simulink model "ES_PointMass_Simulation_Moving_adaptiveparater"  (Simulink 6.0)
settings: Solver=ode45  StartTime=0.0  StopTime=tmax  FixedStep=deltaT  MaxStep=deltaT+.001  MinStep=deltaT-.001  RelTol=1e-3
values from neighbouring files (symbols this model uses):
  ax = .05    (= 0.05)    [ES_PointMass_Values.m]    (also in ES_SimplifyPointMass_Values.m; ES_Unstable_Values.m; doublepointmass.m; pointmass.m)
  ay = .05    (= 0.05)    [ES_PointMass_Values.m]    (also in ES_SimplifyPointMass_Values.m; ES_Unstable_Values.m; doublepointmass.m; pointmass.m)
  centx = -1    [ES_PointMass_Values.m]    (also in ES_SimplifyPointMass_Values.m; ES_Unstable_Values.m; doublepointmass.m; pointmass.m)
  centy = -1    [ES_PointMass_Values.m]    (also in ES_SimplifyPointMass_Values.m; ES_Unstable_Values.m; doublepointmass.m; pointmass.m)
  cx = 20    [ES_PointMass_Values.m]    (also in ES_SimplifyPointMass_Values.m = 15; ES_Unstable_Values.m = 15; doublepointmass.m; pointmass.m)
  cy = 20    [ES_PointMass_Values.m]    (also in ES_SimplifyPointMass_Values.m = 15; ES_Unstable_Values.m = 15; doublepointmass.m; pointmass.m)
  ICx = 1    [ES_PointMass_Values.m]    (also in ES_SimplifyPointMass_Values.m; ES_Unstable_Values.m = 0; ES_Unicycle_nc_values_tune_V.m = 1.8; ES_Unicycle_nc_values_tune_V_moving.m = 1.5)
  ICy = 1    [ES_PointMass_Values.m]    (also in ES_SimplifyPointMass_Values.m; ES_Unstable_Values.m = 0; ES_Unicycle_nc_values_tune_V.m = 2; ES_Unicycle_nc_values_tune_V_moving.m = 2)
  omega = 0.1    [ES_PointMass_Values.m]    (also in ES_SimplifyPointMass_Values.m; ES_Unstable_Values.m; ES_Unicycle_Values_SI.m; abs_perturbation.m = x(:,2))
  qx = 1    [ES_PointMass_Values.m]    (also in ES_SimplifyPointMass_Values.m; ES_Unstable_Values.m; ES_Unicycle_nc_values_tune_V.m = 0.5; ES_Unicycle_nc_values_tune_V_moving.m = 0.5)
  qy = 0.5    [ES_PointMass_Values.m]    (also in ES_SimplifyPointMass_Values.m; ES_Unstable_Values.m; ES_Unicycle_nc_values_tune_V.m = 0.25; ES_Unicycle_nc_values_tune_V_moving.m = 0.25)
  root = 1    [ES_PointMass_Values.m]    (also in ES_SimplifyPointMass_Values.m; ES_Unstable_Values.m; doublepointmass.m; pointmass.m)
  tmax = 50    [ES_PointMass_Values.m]    (also in ES_SimplifyPointMass_Values.m = 80; ES_Unstable_Values.m = 20; ES_Unicycle_nc_values_tune_V.m; ES_Unicycle_nc_values_tune_V_moving.m = 300)
  wx = 30    [ES_PointMass_Values.m]    (also in ES_SimplifyPointMass_Values.m; ES_Unstable_Values.m; doublepointmass.m; pointmass.m = 20)
  wy = 30    [ES_PointMass_Values.m]    (also in ES_SimplifyPointMass_Values.m; ES_Unstable_Values.m; doublepointmass.m; pointmass.m = 20)
undefined symbols (not defined in the file or in its folder): Graph, sfunxy, simulink3, Sinks, XY
libraries: simulink x2

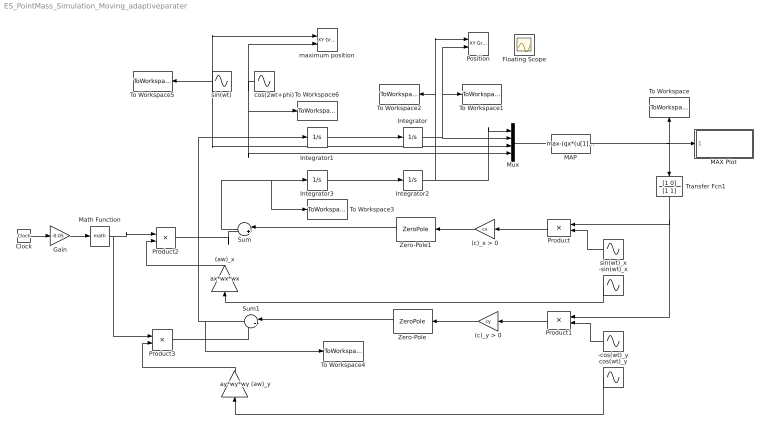
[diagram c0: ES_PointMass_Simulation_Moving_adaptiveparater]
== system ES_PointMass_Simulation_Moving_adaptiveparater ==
  (aw)_x : Gain  Orientation=up  Gain=ax*wx*wx
  (aw)_y : Gain  Orientation=up  Gain=ay*wy*wy
  (c)_x > 0 : Gain  Orientation=left  Gain=cx
  (c)_y > 0 : Gain  Orientation=left  Gain=cy
  -cos(wt)_y : Sin  Orientation=left  Amplitude=-1  Frequency=wy  Phase=pi/2  SampleTime=0
  -sin(wt)_x : Sin  Orientation=left  Frequency=wx  Phase=pi  SampleTime=0
  Clock : Clock
  Floating Scope : Scope  NumInputPorts=2
  Gain : Gain  Gain=-0.05
  Integrator : Integrator  InitialCondition=ICy
  Integrator1 : Integrator
  Integrator2 : Integrator  InitialCondition=ICx
  Integrator3 : Integrator
  MAP : Fcn  Expr=max-(qx*(u[1]-u[3])^2+qy*(u[2]-u[4])^2)^(root)
  MAX Plot : Subsystem
  Math Function : Math
  Mux : Mux
  Position : simulink/Sinks/XY Graph  xmin=centx - abs(0) -2  xmax=centx + abs(0) + 3  ymin=centy - abs(0)-2  ymax=centy + abs(0) + 3  st=-1
  Product : Product  Orientation=left
  Product1 : Product  Orientation=left
  Product2 : Product
  Product3 : Product
  Sum : Sum  Orientation=left  Inputs=|++
  Sum1 : Sum  Orientation=left  Inputs=|++
  To Workspace : ToWorkspace  VariableName=MAX  SampleTime=-1  SaveFormat=Array
  To Workspace1 : ToWorkspace  VariableName=Y  SampleTime=-1  SaveFormat=Array
  To Workspace2 : ToWorkspace  VariableName=X  SampleTime=-1  SaveFormat=Array
  To Workspace3 : ToWorkspace  VariableName=Vx  SampleTime=-1  SaveFormat=Array
  To Workspace4 : ToWorkspace  VariableName=Vy  SampleTime=-1  SaveFormat=Array
  To Workspace5 : ToWorkspace  VariableName=centerx  SampleTime=-1  SaveFormat=Array
  To Workspace6 : ToWorkspace  VariableName=centery  SampleTime=-1  SaveFormat=Array
  Transfer Fcn1 : TransferFcn  Orientation=down  Numerator=[1 0]  Denominator=[1 1]
  Zero-Pole : ZeroPole  Orientation=left  Zeros=[-2]  Poles=[-5]  Gain=[2]
  Zero-Pole1 : ZeroPole  Orientation=left  Zeros=[-2]  Poles=[-5]  Gain=[2]
  cos(2wt+phi) : Sin  Orientation=left  Frequency=2*omega  Phase=3  SampleTime=0
  cos(wt)_y : Sin  Orientation=left  Frequency=wy  Phase=pi/2  SampleTime=0
  maximum position : simulink/Sinks/XY Graph  xmin=centx - abs(0) -2  xmax=centx + abs(0) + 3  ymin=centy - abs(0)-2  ymax=centy + abs(0) + 3  st=-1
  sin(wt) : Sin  Orientation=left  Frequency=omega  SampleTime=0
  sin(wt)_x : Sin  Orientation=left  Frequency=wx  SampleTime=0
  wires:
  Integrator/1 -> To Workspace1/1, Position/2, Mux/2
  Integrator2/1 -> Mux/1, To Workspace2/1, Position/1
  Sum/1 -> Integrator3/1, To Workspace3/1
  sin(wt)_x/1 -> Product/2
  (c)_y > 0/1 -> Zero-Pole/1
  (c)_x > 0/1 -> Zero-Pole1/1
  Product1/1 -> (c)_y > 0/1
  -sin(wt)_x/1 -> (aw)_x/1
  Product/1 -> (c)_x > 0/1
  Sum1/1 -> Integrator1/1, To Workspace4/1
  Mux/1 -> MAP/1
  MAP/1 -> MAX Plot/1(MAX Seeking Value), To Workspace/1, Transfer Fcn1/1
  -cos(wt)_y/1 -> Product1/2
  cos(wt)_y/1 -> (aw)_y/1
  Transfer Fcn1/1 -> Product/1, Product1/1
  Integrator1/1 -> Integrator/1
  Integrator3/1 -> Integrator2/1
  Zero-Pole/1 -> Sum1/1
  Zero-Pole1/1 -> Sum/1
  sin(wt)/1 -> maximum position/1, To Workspace5/1, Mux/3
  cos(2wt+phi)/1 -> maximum position/2, To Workspace6/1, Mux/4
  Product2/1 -> Sum/2
  (aw)_y/1 -> Product3/2
  Product3/1 -> Sum1/2
  (aw)_x/1 -> Product2/2
  Clock/1 -> Gain/1
  Gain/1 -> Math Function/1
  Math Function/1 -> Product2/1, Product3/1

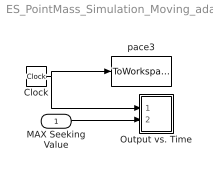
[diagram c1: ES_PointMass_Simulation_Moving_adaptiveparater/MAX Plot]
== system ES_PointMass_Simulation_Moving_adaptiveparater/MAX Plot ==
  MAX Seeking Value : Inport  Port=1  LatchInput=off
  Clock : Clock
  Output vs. Time : Subsystem  AncestorBlock=simulink3/Sinks/XY Graph  LoadFcn=sfunxy([],[],[],'LoadBlock')  StartFcn=sfunxy([],[],[],'Start')  StopFcn=sfunxy([],[],[],'Stop')  TreatAsAtomicUnit=on  SimViewingDevice=on  mask(XY scope.){xmin=0, xmax=tmax, ymin=-3, ymax=max + 2, st=-1}
      mask prompts: xmin "x-min:"; xmax "x-max:"; ymin "y-min:"; ymax "y-max:"; st "Sample time:"
      mask help: XY scope using MATLAB graph window. First input is used as time base. Enter plotting ranges.
  pace3 : ToWorkspace  VariableName=T  SampleTime=-1  SaveFormat=Array
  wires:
  Clock/1 -> pace3/1, Output vs. Time/1(time)
  MAX Seeking Value/1 -> Output vs. Time/2(MAX Seeking Value)

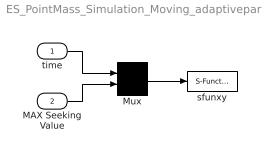
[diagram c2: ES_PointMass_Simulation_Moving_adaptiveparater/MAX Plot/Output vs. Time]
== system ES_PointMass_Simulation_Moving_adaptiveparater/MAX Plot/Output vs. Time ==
  time : Inport  Port=1  LatchInput=off
  MAX Seeking Value : Inport  Port=2  LatchInput=off
  Mux : Mux  Inputs=2
  sfunxy : S-Function  FunctionName=sfunxy  Parameters=[xmin xmax ymin ymax], st
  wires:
  Mux/1 -> sfunxy/1
  time/1 -> Mux/1
  MAX Seeking Value/1 -> Mux/2
